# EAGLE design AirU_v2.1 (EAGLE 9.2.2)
COMPANY: ADAFRUIT INDUSTRIES; DRAWN: KTOWN; REV: B

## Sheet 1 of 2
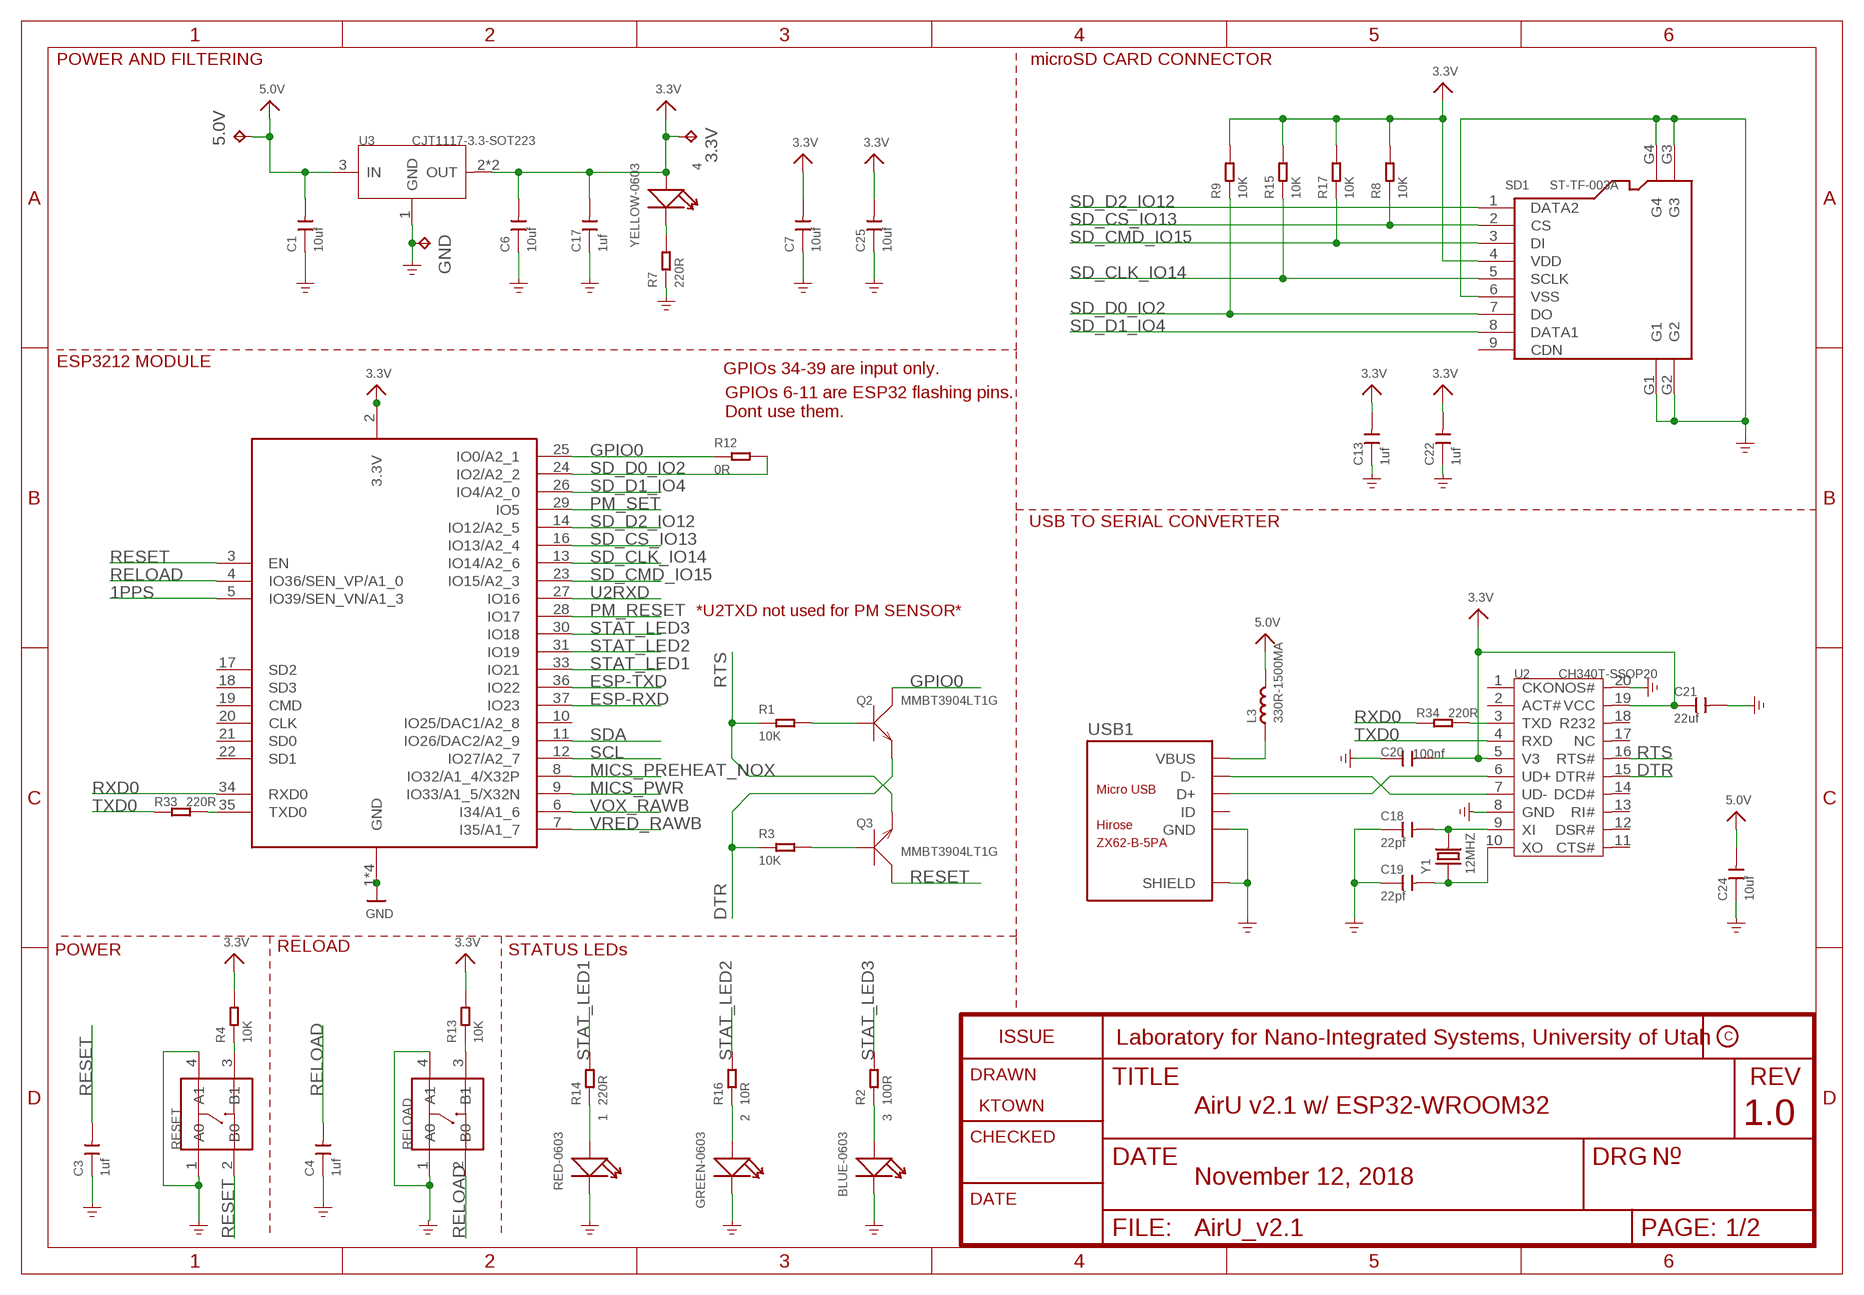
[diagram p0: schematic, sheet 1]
FRAME1 (FRAME_A4): COMPANY: TETRAD: SENSOR NETWORK SOLUTIONS, LLC; REV: 1.0

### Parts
1  RED-0603  LED-SMD-RED-DIFFUSED(0603)  [LED-0603]
2  GREEN-0603  SMD-LED-CLEAR-GREEN(0603)  [LED-0603]
3  BLUE-0603  SMD-LED-CLEAR-BLUE(0603)  [LED-0603]
3.3V  TPTP20SQ  [TP20SQ]
4  YELLOW-0603  SMD-LED-CLEAR-YELLOW(0603)  [LED-0603]
5.0V  TPTP20SQ  [TP20SQ]
C1  10uf  CERAMIC-10UF-10V-10%-X5R(0603)  [C0603]
C3  1uf  CERAMIC-1UF-25V-10%-X7R(0603)  [C0603]
C4  1uf  CERAMIC-1UF-25V-10%-X7R(0603)  [C0603]
C6  10uf  CERAMIC-10UF-10V-10%-X5R(0603)  [C0603]
C7  10uf  CERAMIC-10UF-10V-10%-X5R(0603)  [C0603]
C13  1uf  CERAMIC-1UF-25V-10%-X7R(0603)  [C0603]
C17  1uf  CERAMIC-1UF-25V-10%-X7R(0603)  [C0603]
C18  22pf  CERAMIC-22PF-50V-5%-NPO(0603)  [C0603]
C19  22pf  CERAMIC-22PF-50V-5%-NPO(0603)  [C0603]
C20  100nf  CERAMIC-100NF-50V-10%-X7R(0603)  [C0603]
C21  22uf  CERAMIC-22UF-6.3V-20%-X5R(0805)  [C0805]
C22  1uf  CERAMIC-1UF-25V-10%-X7R(0603)  [C0603]
C24  10uf  CERAMIC-10UF-10V-10%-X5R(0603)  [C0603]
C25  10uf  CERAMIC-10UF-10V-10%-X5R(0603)  [C0603]
GND  TPTP20SQ  [TP20SQ]
L3  330R-1500MA  SMD-FERRITE-BEAD-330R-1500MA(0805)'0805'  [L0805]
Q2  MMBT3904LT1G  SMD-TRANSISTORS-NPN-40V-200MA-MMBT3904LT1G(SOT-23)  [SOT-23]
Q3  MMBT3904LT1G  SMD-TRANSISTORS-NPN-40V-200MA-MMBT3904LT1G(SOT-23)  [SOT-23]
R1  10K  SMD-RES-10K-1%-1/10W(0603)  [R0603]
R2  100R  SMD-RES-100R-5%-1/10W(0603)  [R0603]
R3  10K  SMD-RES-10K-1%-1/10W(0603)  [R0603]
R4  10K  SMD-RES-10K-1%-1/10W(0603)  [R0603]
R7  220R  SMD-RES-220R-5%-1/10W(0603)  [R0603]
R8  10K  SMD-RES-10K-1%-1/10W(0603)  [R0603]
R9  10K  SMD-RES-10K-1%-1/10W(0603)  [R0603]
R12  0R  SMD-RES-0R-5%-1/10W(0603)  [R0603]
R13  10K  SMD-RES-10K-1%-1/10W(0603)  [R0603]
R14  220R  SMD-RES-220R-5%-1/10W(0603)  [R0603]
R15  10K  SMD-RES-10K-1%-1/10W(0603)  [R0603]
R16  10R  SMD-RES-10R-5%-1/10W(0603)  [R0603]
R17  10K  SMD-RES-10K-1%-1/10W(0603)  [R0603]
R33  220R  SMD-RES-220R-5%-1/10W(0603)  [R0603]
R34  220R  SMD-RES-220R-5%-1/10W(0603)  [R0603]
RELOAD  DIP-SWITCH-TACTILE-SPST-NO/TS-1109(4P-D6.0MM)'TS-1109'  [SW4-6.0X6.0X5.0MM]
RESET  DIP-SWITCH-TACTILE-SPST-NO/TS-1109(4P-D6.0MM)'TS-1109'  [SW4-6.0X6.0X5.0MM]
SD1  ST-TF-003A  MICRO-SD-CARD-SOCKET-9P(ST-TF-003A)  [MICRO-SD9+4P-SMD-16.1X14.5X1.85MM]
U2  CH340T-SSOP20  INTERFACE-CH340T(SSOP20)  [SSOP20-0.65-7.6X5.2MM]
U3  CJT1117-3.3-SOT223  PMIC-CJT1117-3.3(SOT223)  [SOT-223]
U7  ESP32_WROOM32_SKINNY  [WROOM32_SKINNY]
USB1  ZX62-B-5PA  MICRO-USB-SMD(ZX62-B-5PA)  [MICRO-USB5+6P-SMD-0.65-AB]
Y1  12MHZ  SMD-CRYSTAL-12MHZ-20PF-20PPM-40R(2P-5.0X3.2MM)  [X2-SMD-5.0X3.2X1.3MM]

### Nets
1PPS: U7.5(IO39/SEN_VN/A1_3) ; also sheet 2
3.3V: 3.3V.TP 4.+ C6.2 C7.2 C13.2 C17.2 C20.2 C21.1 C22.2 C25.2 R4.2 R8.2 R9.2 R13.2 R15.2 R17.2 SD1.4(VDD) U2.5(V3) U2.19(VCC) U3.2(OUT) U3.TER(OUT) U7.2(3.3V) ; also sheet 2
5.0V: 5.0V.TP C1.2 C24.2 L3.2 U3.3(IN) ; also sheet 2
DTR: Q2.2(E) R3.1 U2.15(DTR#)
ESP-RXD: U7.37(IO23) ; also sheet 2
ESP-TXD: U7.36(IO22) ; also sheet 2
GND: 1.- 2.- 3.- C1.1 C3.1 C4.1 C6.1 C7.1 C13.1 C17.1 C18.1 C19.1 C20.1 C21.2 C22.1 C24.1 C25.1 GND.TP R7.1 RELOAD.1(A0) RELOAD.4(A1) RESET.1(A0) RESET.4(A1) SD1.6(VSS) SD1.G1 SD1.G2 SD1.G3 SD1.G4 U2.8(GND) U2.20(NOS#) U3.1(GND) U7.1(GND) U7.15(GND) U7.38(GND) U7.P$1(GND) USB1.5(GND) USB1.P1(SHIELD) USB1.P2(SHIELD) USB1.P3_1(SHIELD) USB1.P3_2(SHIELD) USB1.P3_3(SHIELD) USB1.P4_1(SHIELD) USB1.P4_2(SHIELD) USB1.P4_3(SHIELD) USB1.P5(SHIELD) USB1.P6(SHIELD) ; supply symbol labelled GND_POWER ; also sheet 2
GPIO0: Q2.3(C) R12.1 U7.25(IO0/A2_1)
MICS_PREHEAT_NOX: U7.8(IO32/A1_4/X32P) ; also sheet 2
MICS_PWR: U7.9(IO33/A1_5/X32N) ; also sheet 2
N$1: 2.+ R16.1
N$7: 1.+ R14.1
N$12: Q3.1(B) R3.2
N$13: Q2.1(B) R1.2
N$22: 3.+ R2.1
N$25: 4.- R7.2
N$26: U2.7(UD-) USB1.2(D-)
N$27: U2.6(UD+) USB1.3(D+)
N$28: C18.2 U2.9(XI) Y1.2
N$29: C19.2 U2.10(XO) Y1.1
N$30: R34.2 U2.3(TXD)
N$33: R33.2 U7.35(TXD0)
N$37: R13.1 RELOAD.3(B1)
N$38: R4.1 RESET.3(B1)
PM_RESET: U7.28(IO17) ; also sheet 2
PM_SET: U7.29(IO5) ; also sheet 2
RELOAD: C4.2 RELOAD.2(B0) U7.4(IO36/SEN_VP/A1_0)
RESET: C3.2 Q3.3(C) RESET.2(B0) U7.3(EN)
RTS: Q3.2(E) R1.1 U2.16(RTS#)
RXD0: R34.1 U7.34(RXD0)
SCL: U7.12(IO27/A2_7) ; also sheet 2
SD_CLK_IO14: R15.1 SD1.5(SCLK) U7.13(IO14/A2_6)
SD_CMD_IO15: R17.1 SD1.3(DI) U7.23(IO15/A2_3)
SD_CS_IO13: R8.1 SD1.2(CS) U7.16(IO13/A2_4)
SD_D0_IO2: R9.1 R12.2 SD1.7(DO) U7.24(IO2/A2_2)
SD_D1_IO4: SD1.8(DATA1) U7.26(IO4/A2_0)
SD_D2_IO12: SD1.1(DATA2) U7.14(IO12/A2_5)
SDA: U7.11(IO26/DAC2/A2_9) ; also sheet 2
STAT_LED1: R14.2 U7.33(IO21)
STAT_LED2: R16.2 U7.31(IO19)
STAT_LED3: R2.2 U7.30(IO18)
TXD0: R33.1 U2.4(RXD)
U2RXD: U7.27(IO16) ; also sheet 2
VBUS: L3.1 USB1.1(VBUS)
VOX_RAWB: U7.6(I34/A1_6) ; also sheet 2
VRED_RAWB: U7.7(I35/A1_7) ; also sheet 2
Unconnected: SD1.9(CDN) U2.1(CKO) U2.2(ACT#) U2.11(CTS#) U2.12(DSR#) U2.13(RI#) U2.14(DCD#) U2.17(NC) U2.18(R232) U7.10(IO25/DAC1/A2_8) U7.17(SD2) U7.18(SD3) U7.19(CMD) U7.20(CLK) U7.21(SD0) U7.22(SD1) USB1.4(ID)

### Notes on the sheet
- POWER AND FILTERING | microSD CARD CONNECTOR
- ESP3212 MODULE
- GPIOs 34-39 are input only.
- GPIOs 6-11 are ESP32 flashing pins.
  Dont use them.
- USB TO SERIAL CONVERTER
- *U2TXD not used for PM SENSOR*
- POWER | RELOAD | STATUS LEDs
- Laboratory for Nano-Integrated Systems, University of Utah
- AirU v2.1 w/ ESP32-WROOM32
- November 12, 2018

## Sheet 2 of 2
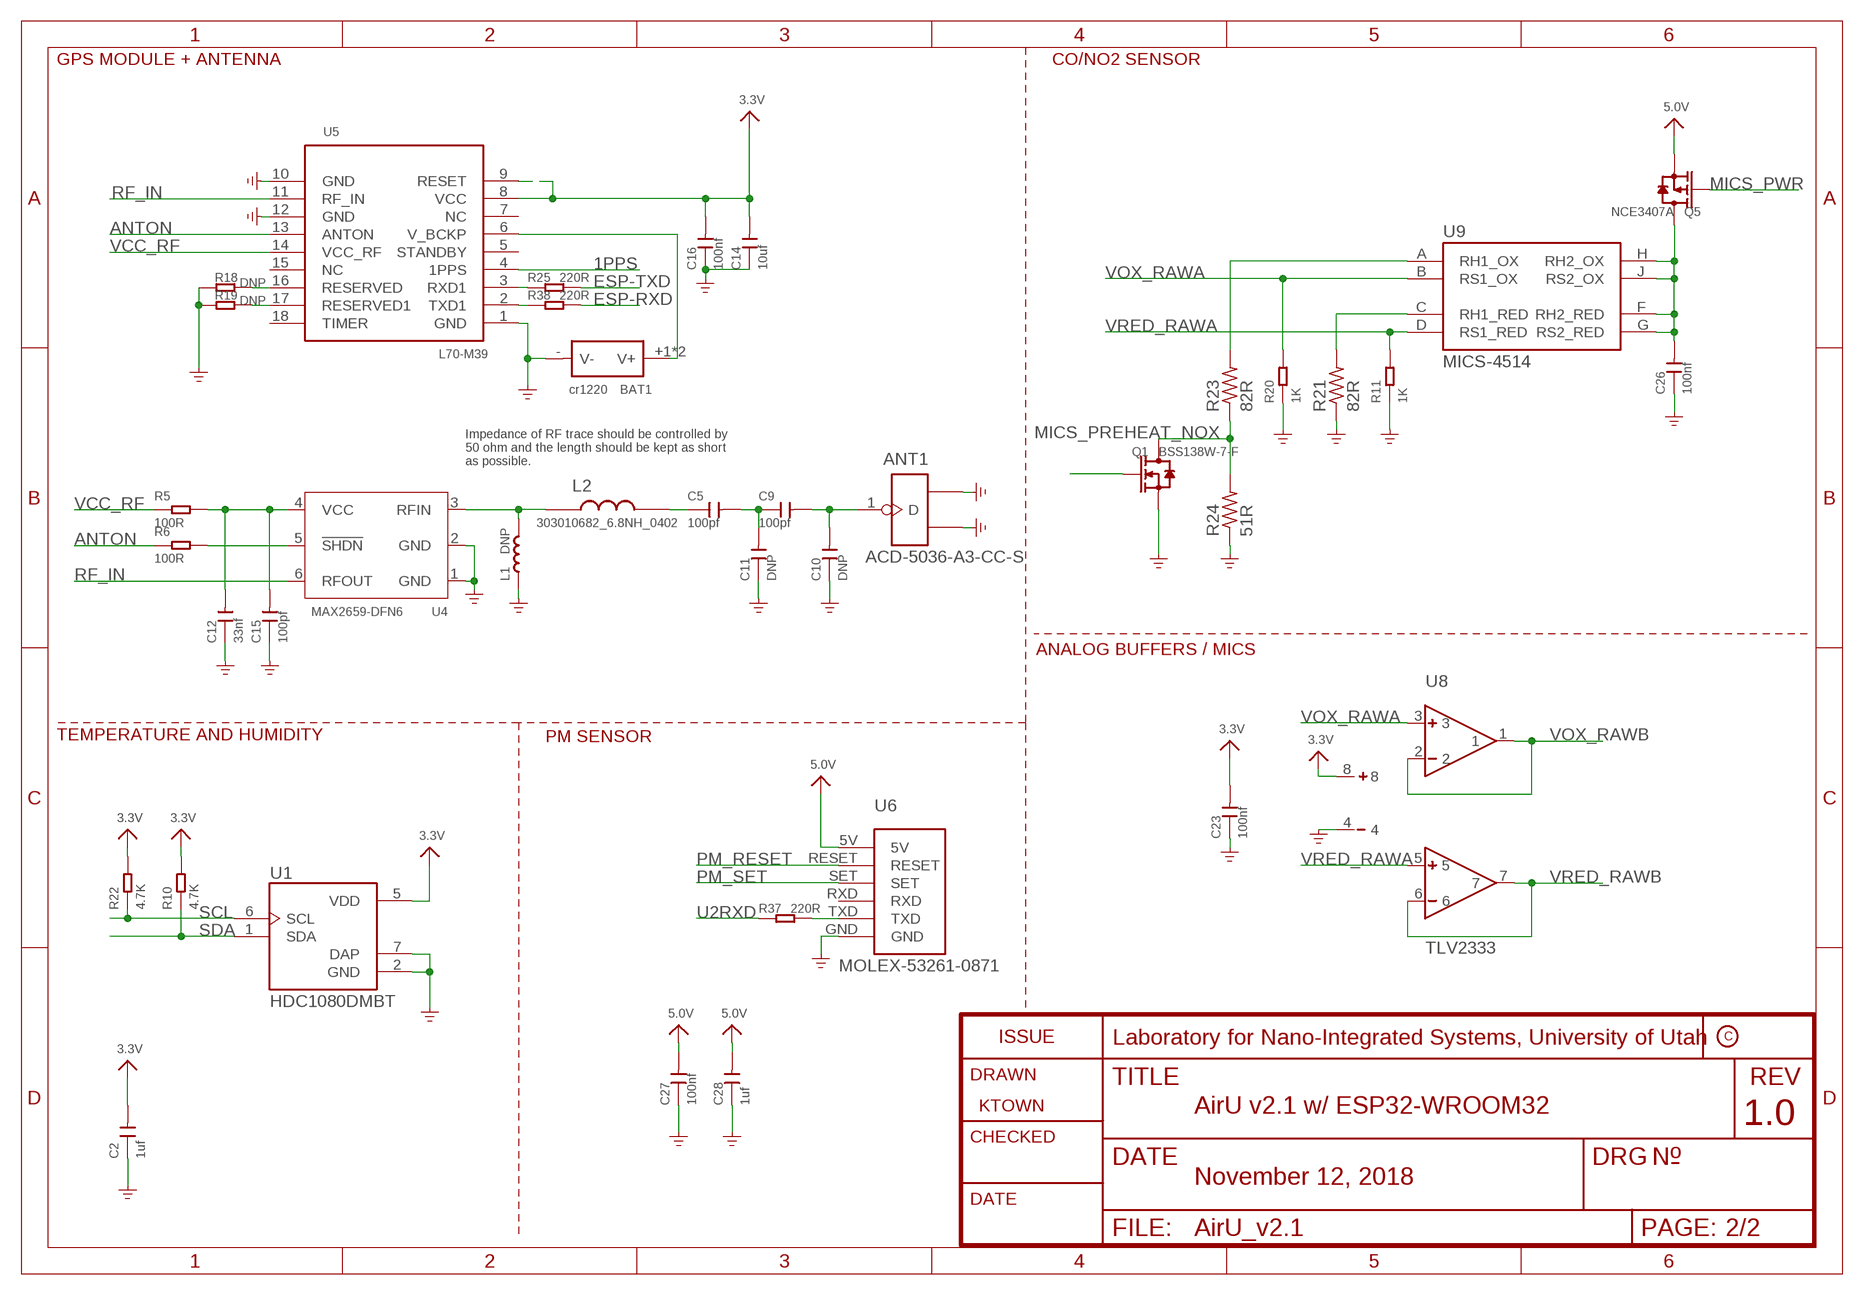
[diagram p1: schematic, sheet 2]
FRAME2 (FRAME_A4): COMPANY: TETRAD: SENSOR NETWORK SOLUTIONS, LLC; REV: 1.0
FRAME3 (FRAME_A4): COMPANY: TETRAD: SENSOR NETWORK SOLUTIONS, LLC; REV: 1.0

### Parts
ANT1  ACD-5036-A3-CC-S  ANTENNA-ACD5036  [ANT3-SMD-5.2X3.7X0.7MM]
BAT1  cr1220  DIP-BATTERY-CELL-HOLDER(1220)  [BAT2P-13.5-CR1220]
C2  1uf  CERAMIC-1UF-25V-10%-X7R(0603)  [C0603]
C5  100pf  CERAMIC-100PF-50V-5%-NPO(0603)  [C0603]
C9  100pf  CERAMIC-100PF-50V-5%-NPO(0603)  [C0603]
C10  DNP  CERAMIC-100PF-50V-5%-NPO(0603)  [C0603]
C11  DNP  CERAMIC-100PF-50V-5%-NPO(0603)  [C0603]
C12  33nf  CERAMIC-33NF-50V-10%-X7R(0603)  [C0603]
C14  10uf  CERAMIC-10UF-10V-10%-X5R(0603)  [C0603]
C15  100pf  CERAMIC-100PF-50V-5%-NPO(0603)  [C0603]
C16  100nf  CERAMIC-100NF-50V-10%-X7R(0603)  [C0603]
C23  100nf  CERAMIC-100NF-50V-10%-X7R(0603)  [C0603]
C26  100nf  CERAMIC-100NF-50V-10%-X7R(0603)  [C0603]
C27  100nf  CERAMIC-100NF-50V-10%-X7R(0603)  [C0603]
C28  1uf  CERAMIC-1UF-25V-10%-X7R(0603)  [C0603]
L1  DNP  INDUCTOR/FERRITE-BEAD-0201  [L0201]
L2  303010682_6.8NH_0402  [L0402]
Q1  BSS138W-7-F  SMD-MOSFET-N-CH-50V-200MA-BSS138W-7-F(SOT-23)  [SOT-23]
Q5  NCE3407A  SMD-MOSFET-P-CH-VDC=30V-ID=4.3A-NCE3407A(SOT-23)  [SOT-23]
R5  100R  SMD-RES-100R-5%-1/10W(0603)  [R0603]
R6  100R  SMD-RES-100R-5%-1/10W(0603)  [R0603]
R10  4.7K  SMD-RES-4.7K-5%-1/10W(0603)  [R0603]
R11  1K  SMD-RES-1K-1%-1/10W(0603)  [R0603]
R18  DNP  SMD-RES-10K-1%-1/10W(0603)  [R0603]
R19  DNP  SMD-RES-10K-1%-1/10W(0603)  [R0603]
R20  1K  SMD-RES-1K-1%-1/10W(0603)  [R0603]
R21  82R  R-US_R0603  [R0603]
R22  4.7K  SMD-RES-4.7K-5%-1/10W(0603)  [R0603]
R23  82R  R-US_R0603  [R0603]
R24  51R  R-US_R0603  [R0603]
R25  220R  SMD-RES-220R-5%-1/10W(0603)  [R0603]
R37  220R  SMD-RES-220R-5%-1/10W(0603)  [R0603]
R38  220R  SMD-RES-220R-5%-1/10W(0603)  [R0603]
U1  HDC1080DMBT  [SON100P300X300X80-7N]
U4  MAX2659-DFN6  AMPLIFIER-MAX2659  [DFN6-0.5-1.5X1.2X0.72MM]
U5  L70-M39  MOUDLE-GPS-L70-HARDWARE  [LGA18-1.1-9.7X10.1X2.5MM]
U6  MOLEX-53261-0871  [MOLEX-53261-0871]
U8  TLV2333  [TLV2333]
U9  MICS-4514  [MICS_10-SMD]

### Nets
1PPS: U5.4(1PPS) ; also sheet 1
3.3V: C2.2 C14.2 C16.2 C23.2 R10.2 R22.2 U1.5(VDD) U5.8(VCC) U5.9(RESET) U8.8 ; also sheet 1
5.0V: C27.2 C28.2 Q5.2(S) U6.5V ; also sheet 1
ANTON: R6.1 U5.13(ANTON)
ESP-RXD: R38.2 ; also sheet 1
ESP-TXD: R25.2 ; also sheet 1
GND: ANT1.2(GND1) ANT1.3(GND2) BAT1.-(V-) C2.1 C10.1 C11.1 C12.1 C14.1 C15.1 C16.1 C23.1 C26.1 C27.1 C28.1 L1.1 Q1.2(S) R11.1 R18.1 R19.1 R20.1 R21.1 R24.1 U1.2(GND) U1.7(DAP) U4.1(GND) U4.2(GND) U5.1(GND) U5.10(GND) U5.12(GND) U6.GND U8.4 ; supply symbol labelled GND_POWER ; also sheet 1
MICS_PREHEAT_NOX: Q1.1(G) ; also sheet 1
MICS_PWR: Q5.1(G) ; also sheet 1
N$2: R21.2 U9.C(RH1_RED)
N$3: C5.2 C9.1 C11.2
N$4: ANT1.1(D) C9.2 C10.2
N$5: L1.2 L2.P$1 U4.3(RFIN)
N$6: R23.2 U9.A(RH1_OX)
N$8: C5.1 L2.P$2
N$9: R6.2 U4.5(!SHDN)
N$10: C12.2 C15.2 R5.2 U4.4(VCC)
N$11: R18.2 U5.16(RESERVED)
N$14: R19.2 U5.17(RESERVED1)
N$23: Q1.3(D) R23.1 R24.2
N$24: C26.2 Q5.3(D) U9.F(RH2_RED) U9.G(RS2_RED) U9.H(RH2_OX) U9.J(RS2_OX)
N$36: R37.2 U6.TXD
PM_RESET: U6.RESET ; also sheet 1
PM_SET: U6.SET ; also sheet 1
RF_IN: U4.6(RFOUT) U5.11(RF_IN)
SCL: R22.1 U1.6(SCL) ; also sheet 1
SDA: R10.1 U1.1(SDA) ; also sheet 1
U1RXD: R25.1 U5.3(RXD1)
U1TXD: R38.1 U5.2(TXD1)
U2RXD: R37.1 ; also sheet 1
V_BCKP: BAT1.+1(V+) BAT1.+2(V+) U5.6(V_BCKP)
VCC_RF: R5.1 U5.14(VCC_RF)
VOX_RAWA: R20.2 U8.3 U9.B(RS1_OX)
VOX_RAWB: U8.1 U8.2 ; also sheet 1
VRED_RAWA: R11.2 U8.5 U9.D(RS1_RED)
VRED_RAWB: U8.6 U8.7 ; also sheet 1
Unconnected: U5.5(STANDBY) U5.7(NC) U5.15(NC) U5.18(TIMER) U6.RXD

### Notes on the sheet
- GPS MODULE + ANTENNA | CO/NO2 SENSOR
- Impedance of RF trace should be controlled by 
  50 ohm and the length should be kept as short 
  as possible.
- ANALOG BUFFERS / MICS
- TEMPERATURE AND HUMIDITY | PM SENSOR
- Laboratory for Nano-Integrated Systems, University of Utah
- AirU v2.1 w/ ESP32-WROOM32
- November 12, 2018

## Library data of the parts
1 = Seeed-LED:LED-SMD-RED-DIFFUSED(0603): 304090042; MPN: 19-217-R6C-AL1M2VY-3T
2 = Seeed-LED:SMD-LED-CLEAR-GREEN(0603): 304090043; MPN: 19-217-G7C-AN1P2-3T
3 = Seeed-LED:SMD-LED-CLEAR-BLUE(0603): 304090045; MPN: 19-217-BHC-ZL1M2RY-3T
3.3V 5.0V GND = testpad:TP: Test pad
4 = Seeed-LED:SMD-LED-CLEAR-YELLOW(0603): 304090044; MPN: 19-217-Y5C-AM1N1VY-3T
ANT1 = Connector-new:ANTENNA-ACD5036; MPN: ACD-5036-A3-CC-S
BAT1 = Seeed-Connector:DIP-BATTERY-CELL-HOLDER(1220): 320170002
C1 C6 C7 C14 C24 C25 = Seeed-Capacitor:CERAMIC-10UF-10V-10%-X5R(0603): 302010103; MPN: CC0603KRX5R6BB106
C2-C4 C13 C17 C22 C28 = Seeed-Capacitor:CERAMIC-1UF-25V-10%-X7R(0603): 302010139; MPN: CC0603KRX7R8BB105
C5 C9 C15 = Seeed-Capacitor:CERAMIC-100PF-50V-5%-NPO(0603): 302010076; MPN: CC0603JRNPO9BN101
C10 C11 = Seeed-Capacitor:CERAMIC-100PF-50V-5%-NPO(0603): 302010076; MPN: CC0603JRNPO9BN101; VALUE: 100pf
C12 = Seeed-Capacitor:CERAMIC-33NF-50V-10%-X7R(0603): 302010088; MPN: CC0603KRX7R9BB333
C16 C20 C23 C26 C27 = Seeed-Capacitor:CERAMIC-100NF-50V-10%-X7R(0603): 302010138; MPN: CC0603KRX7R9BB104
C18 C19 = Seeed-Capacitor:CERAMIC-22PF-50V-5%-NPO(0603): 302010143; MPN: CC0603JRNPO9BN220
C21 = Seeed-Capacitor:CERAMIC-22UF-6.3V-20%-X5R(0805): 302010171; MPN: CC0805MKX5R5BB226
L1 = Discrete-new:INDUCTOR/FERRITE-BEAD
L2 = Seeed-OPL-2017-01-Inductor-Akita:303010682_6.8NH_0402: Murata;LQW15AN6N8G00D, SMD Inductor 6.8nH-2%-700mA;0402, SKU: 303010682
L3 = Seeed-Inductor:SMD-FERRITE-BEAD-330R-1500MA(0805): 303030006; MPN: BLM21PG331SN1D
Q1 = Seeed-Transistor:SMD-MOSFET-N-CH-50V-200MA-BSS138W-7-F(SOT-23): 305030000; MPN: BSS138W-7-F
Q2 Q3 = Seeed-Transistor:SMD-TRANSISTORS-NPN-40V-200MA-MMBT3904LT1G(SOT-23): 305010013; MPN: MMBT3904LT1G
Q5 = Seeed-Transistor:SMD-MOSFET-P-CH-VDC=30V-ID=4.3A-NCE3407A(SOT-23): 305030010; MPN: NCE3407A
R1 R3 R4 R8 R9 R13 R15 R17 = Seeed-Resistor:SMD-RES-10K-1%-1/10W(0603): 301010299; MPN: RC0603FR-0710KL
R2 R5 R6 = Seeed-Resistor:SMD-RES-100R-5%-1/10W(0603): 301010090; MPN: RC0603JR-07100RL
R7 R14 R25 R33 R34 R37 R38 = Seeed-Resistor:SMD-RES-220R-5%-1/10W(0603): 301010163; MPN: RC0603JR-07220RL
R10 R22 = Seeed-Resistor:SMD-RES-4.7K-5%-1/10W(0603): 301010290; MPN: RC0603JR-074K7L
R11 R20 = Seeed-Resistor:SMD-RES-1K-1%-1/10W(0603): 301010298; MPN: RC0603FR-071KL
R12 = Seeed-Resistor:SMD-RES-0R-5%-1/10W(0603): 301010292; MPN: RC0603JR-070RL
R16 = Seeed-Resistor:SMD-RES-10R-5%-1/10W(0603): 301010096; MPN: RC0603JR-0710RL
R18 R19 = Seeed-Resistor:SMD-RES-10K-1%-1/10W(0603): 301010299; MPN: RC0603FR-0710KL; VALUE: 10K
R21 R23 R24 = rcl:R-US_: RESISTOR, American symbol; SPICEPREFIX: R
RELOAD RESET = Seeed-Switch:DIP-SWITCH-TACTILE-SPST-NO/TS-1109(4P-D6.0MM): 311020024
SD1 = Seeed-Connector:MICRO-SD-CARD-SOCKET-9P(ST-TF-003A): 320090000; MPN: ST-TF-003A
U1 = HDC1080DMBT_TITempHum:HDC1080DMBT: HDC1080 Low Power, High Accuracy Digital Humidity Sensor with Temperature Sensor 6-WSON -40 to 125; DESCRIPTION: HDC1080 Low Power, High Accuracy Digital Humidity Sensor with Temperature Sensor 6-WSON -40 to 125; DIGI-KEY_PART_NUMBER: 296-43864-1-ND; DIGI-KEY_PURCHASE_URL: https://www.digikey.com/product-detail/en/texas-instruments/HDC1080DMBT/296-43864-1-ND/5878615?utm_source=snapeda&utm_medium=aggregator&utm_campaign=symbol; MF: Texas Instruments; MP: HDC1080DMBT; PACKAGE: WDFN-6 Texas Instruments
U2 = Seeed-IC:INTERFACE-CH340T(SSOP20): 310070026; MPN: CH340T
U3 = Seeed-IC:PMIC-CJT1117-3.3(SOT223): 310030097; MPN: CJT1117-3.3
U4 = IC-new:AMPLIFIER-MAX2659: GPS/GNSS Low-Noise Amplifier; MPN: MAX2659
U5 = moudle-new:MOUDLE-GPS-L70-HARDWARE: L70 GPS module; MPN: L70; VALUE: L70
U6 = Molex_53261_0871_Connector:MOLEX-53261-0871
U7 = microbuilder:ESP32_WROOM32
U8 = tlv2333:TLV2333
U9 = MICS-4514:MICS-4514: Metal oxide MEMS carbon monoxide (CO) and NOx sensor in an SMD package.; AVAILABILITY: Unavailable; MF: Amphenol; MP: MICS-4514; PACKAGE: None; PRICE: 11.82 USD
USB1 = Seeed-Connector:MICRO-USB-SMD(ZX62-B-5PA): 320010005; MPN: ZX62-B-5PA
Y1 = Seeed-Crystal Oscillator:SMD-CRYSTAL-12MHZ-20PF-20PPM-40R(2P-5.0X3.2MM): 306010047; MPN: 5032/2P

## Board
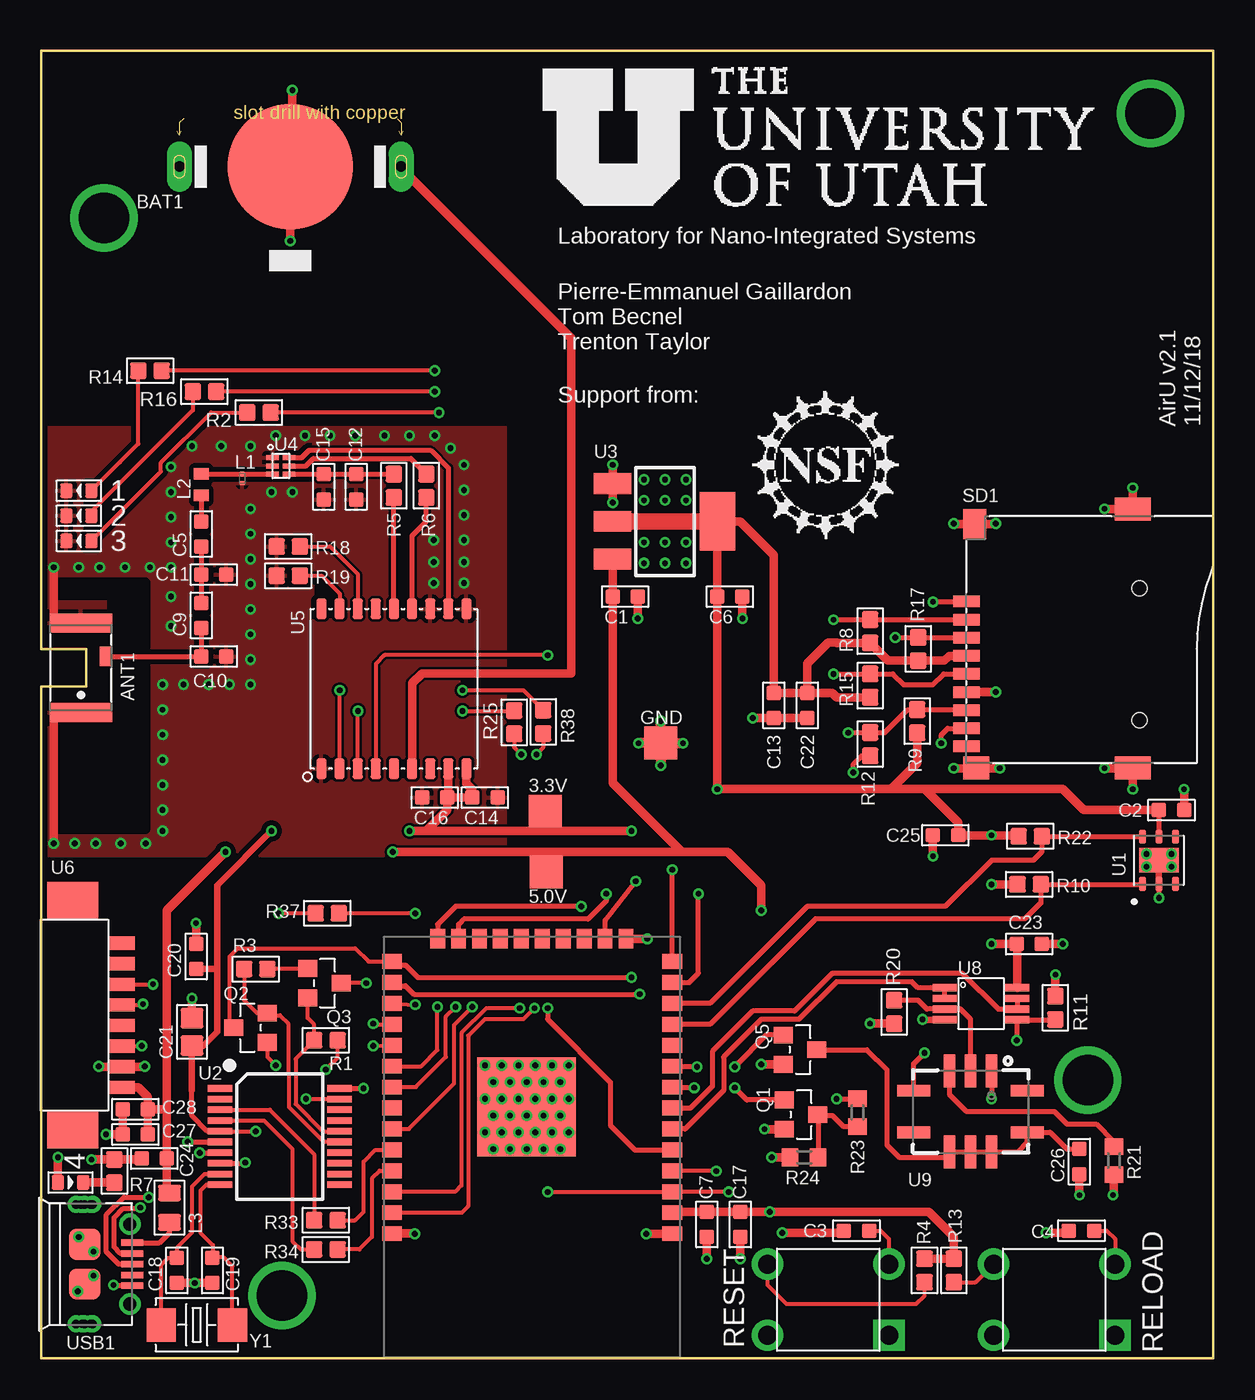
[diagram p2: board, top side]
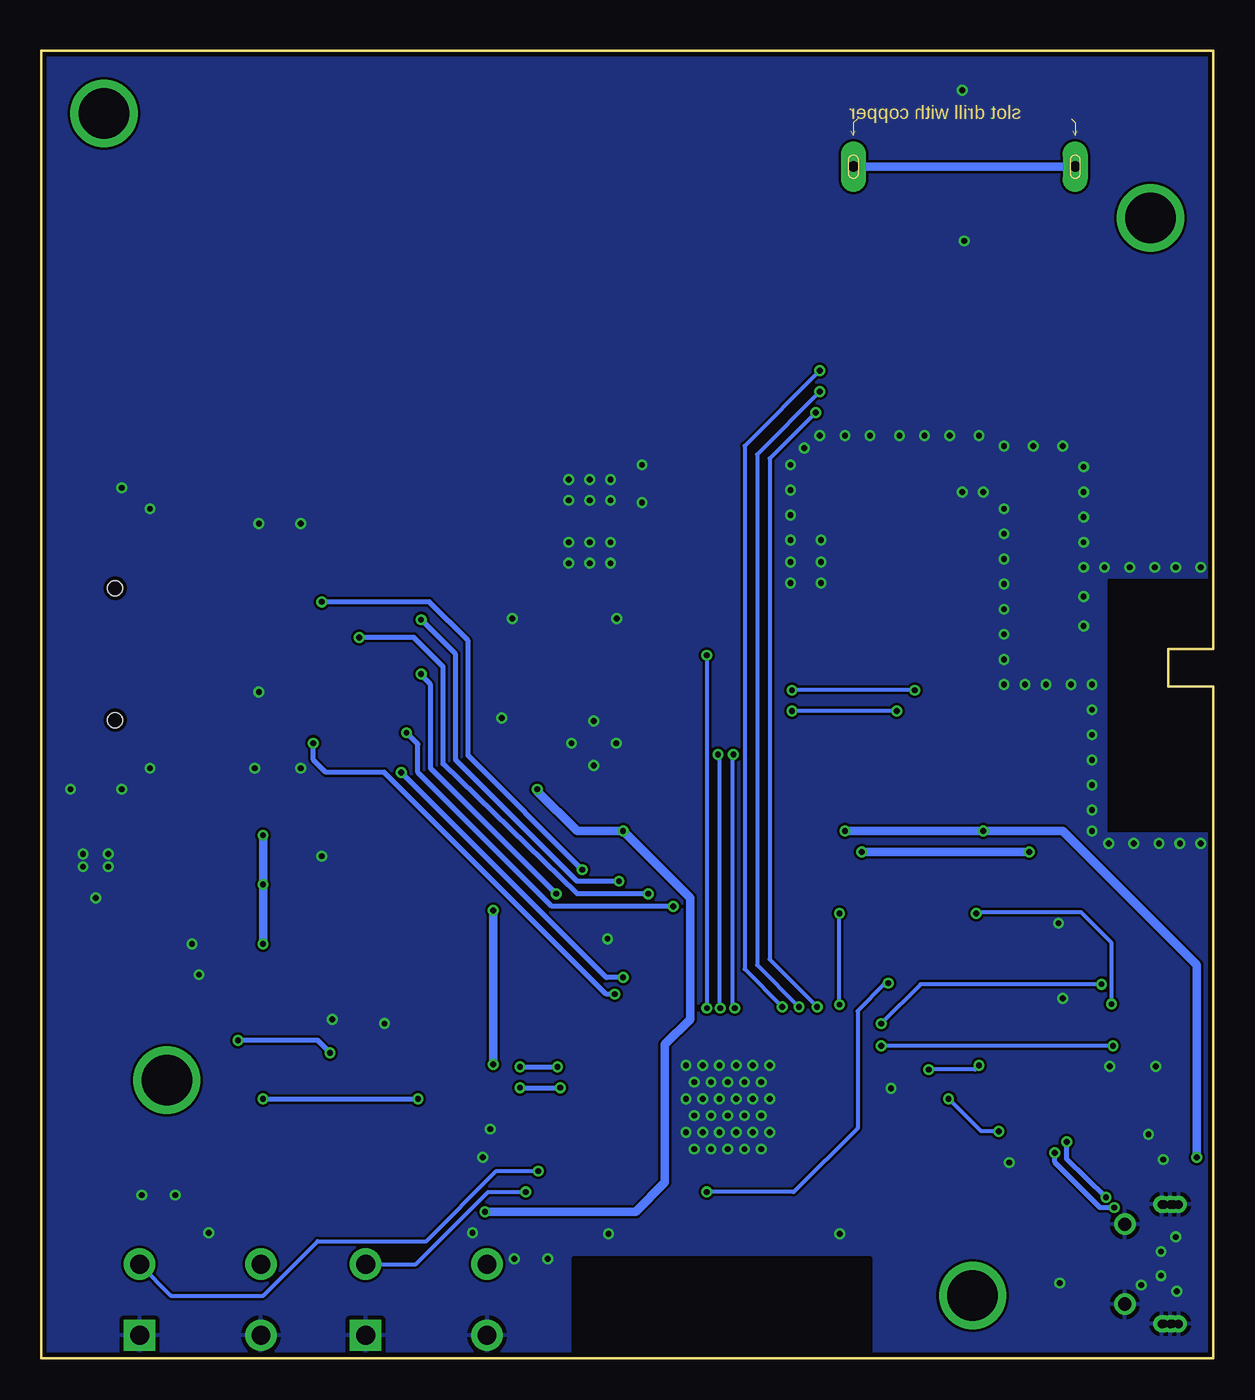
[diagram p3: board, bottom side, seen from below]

Size 71.12 x 79.38 mm. Coordinates in mm from the lower left corner, seen from the top.
Outline: 0,0 71.12,0 71.12,79.38 0,79.38 0,43.05 2.73,43.05 2.73,40.77 0,40.77 0,0
Copper layers (1*16): Top 0.035mm / dielectric 1.5mm / Bottom 0.035mm
Design rules "SeeedStudio_2layer_DRU_no_angle_20140221": minimum track width 6mil, minimum drill 12mil, track to track 6mil, track to pad 6mil, pad to pad 6mil, via to via 6mil, smd to smd 0mil, copper to edge 10mil, drill to drill 10mil, minimum pad ring 10mil, minimum via ring 6mil, stop-mask expansion 2mil, vias tented up to drill 100mil, thermal gap 10mil
tRestrict: area 20.8,0.1 to 38.8,6.1
bRestrict: area 20.8,0.1 to 38.8,6.1; area 0,32.1 to 6.3,47.1; area 0,32 to 6.3,47.2

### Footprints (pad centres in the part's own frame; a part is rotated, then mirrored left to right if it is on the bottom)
LED-0603 = smd 0.762 x 0.889: + -0.762,0; - 0.762,0
TP20SQ = smd 2 x 2: TP 0,0
ANT3-SMD-5.2X3.7X0.7MM = smd 0.75 x 1.2: 1 1.525,0.7 | smd 3.8 x 1.15: 2 0,2.725; 3 0,-2.725
BAT2P-13.5-CR1220 = drill 0.635 pad 1.524 long: +1 6.731,0; +2 -6.731,0 | smd 7.62 x 7.62: - 0,0
C0603 = smd 0.889 x 0.889: 1 0,0.762; 2 0,-0.762
C0805 = smd 1.397 x 1.27: 1 0,0.835; 2 0,-0.835
L0201 = smd 0.279 x 0.318: 1 -0.279,0; 2 0.279,0
L0402 = smd 0.7 x 0.9: P$1 -0.65,0; P$2 0.65,0
L0805 = smd 1.016 x 1.397: 1 -0.889,0; 2 0.889,0
SOT-23 = smd 1.016 x 1.143: 1 -0.889,-1.016; 2 0.889,-1.016; 3 0,1.016
R0603 = smd 1.016 x 1.016: 1 0,0.708; 2 0,-0.708
R0603' = smd 1 x 1.1: 1 -0.85,0; 2 0.85,0
SW4-6.0X6.0X5.0MM = drill 1.143 pad 1.905 square: 1 -3.683,2.159 | drill 1.143 pad 1.905: 2 -3.683,-2.159; 3 3.683,-2.159; 4 3.683,2.159
MICRO-SD9+4P-SMD-16.1X14.5X1.85MM = smd 1.6 x 0.7: 1 0,2.25; 2 0,1.15; 3 0,0.05; 4 0,-1.05; 5 0,-2.15; 6 0,-3.25; 7 0,-4.35; 8 0,-5.45; 9 0,-6.55 | smd 1.6 x 1.4: G1 0.6,-7.85 | smd 2.2 x 1.4: G2 10.1,-7.85; G3 10.1,7.85 | smd 1.4 x 1.8: G4 0.5,6.95 | hole 0.9: 10.5,-4.95; 10.5,3.05
SON100P300X300X80-7N = smd 0.86 x 0.42: 1 -1.435,1; 2 -1.435,0; 3 -1.435,-1; 4 1.435,-1; 5 1.435,0; 6 1.435,1 | smd 1.5 x 2.4: 7 0,0
SSOP20-0.65-7.6X5.2MM = smd 0.4 x 1.5: 1 -2.925,-3.625; 2 -2.275,-3.625; 3 -1.625,-3.625; 4 -0.975,-3.625; 5 -0.325,-3.625; 6 0.325,-3.625; 7 0.975,-3.625; 8 1.625,-3.625; 9 2.275,-3.625; 10 2.925,-3.625; 11 2.925,3.625; 12 2.275,3.625; 13 1.625,3.625; 14 0.975,3.625; 15 0.325,3.625; 16 -0.325,3.625; 17 -0.975,3.625; 18 -1.625,3.625; 19 -2.275,3.625; 20 -2.925,3.625
SOT-223 = smd 1.27 x 2.286: 1 -2.286,-3.175; 2 0,-3.175; 3 2.286,-3.175 | smd 3.556 x 2.159: TER 0,3.175
DFN6-0.5-1.5X1.2X0.72MM = smd 0.3 x 0.75: 1 -0.5,-0.5; 2 0,-0.5; 3 0.5,-0.5; 4 0.5,0.5; 5 0,0.5; 6 -0.5,0.5
LGA18-1.1-9.7X10.1X2.5MM = smd 1.27 x 0.635: 1 4.85,-4.4; 2 4.85,-3.3; 3 4.85,-2.2; 4 4.85,-1.1; 5 4.85,0; 6 4.85,1.1; 7 4.85,2.2; 8 4.85,3.3; 9 4.85,4.4; 10 -4.85,4.4; 11 -4.85,3.3; 12 -4.85,2.2; 13 -4.85,1.1; 14 -4.85,0; 15 -4.85,-1.1; 16 -4.85,-2.2; 17 -4.85,-3.3; 18 -4.85,-4.4
MOLEX-53261-0871 = smd 0.8 x 1.6: 5V 4.375,0.8; GND 3.125,0.8; NC@1 -4.375,0.8; NC@2 -3.125,0.8; RESET -1.875,0.8; RXD 0.625,0.8; SET 1.875,0.8; TXD -0.625,0.8 | smd 2.2 x 3.1: NC@3 -6.975,-2.16; NC@4 6.975,-2.16
WROOM32_SKINNY = smd 1.2 x 0.9: 1 -8.5,5; 2 -8.5,3.73; 3 -8.5,2.46; 4 -8.5,1.19; 5 -8.5,-0.08; 6 -8.5,-1.35; 7 -8.5,-2.62; 8 -8.5,-3.89; 9 -8.5,-5.16; 10 -8.5,-6.43; 11 -8.5,-7.7; 12 -8.5,-8.97; 13 -8.5,-10.24; 14 -8.5,-11.51; 25 8.5,-11.51; 26 8.5,-10.24; 27 8.5,-8.97; 28 8.5,-7.7; 29 8.5,-6.43; 30 8.5,-5.16; 31 8.5,-3.89; 32 8.5,-2.62; 33 8.5,-1.35; 34 8.5,-0.08; 35 8.5,1.19; 36 8.5,2.46; 37 8.5,3.73; 38 8.5,5 | smd 0.9 x 1.2: 15 -5.7,-12.9; 16 -4.43,-12.9; 17 -3.16,-12.9; 18 -1.89,-12.9; 19 -0.62,-12.9; 20 0.65,-12.9; 21 1.92,-12.9; 22 3.19,-12.9; 23 4.46,-12.9; 24 5.73,-12.9 | smd 6 x 6: P$1 0.34,-2.7
TLV2333 = smd 1.45 x 0.45: 1 0.725,2.175; 2 0.725,1.525; 3 0.725,0.875; 4 0.725,0.225; 5 5.125,0.225; 6 5.125,0.875; 7 5.125,1.525; 8 5.125,2.175
MICS_10-SMD = smd 0.7 x 2: A 1.27,2.45; B 0,2.45; C -1.27,2.45; F -1.27,-2.45; G 0,-2.45; H 1.27,-2.45 | smd 2 x 0.7: D -3.45,1.27; E -3.45,-1.27; J 3.45,-1.27; K 3.45,1.27
MICRO-USB5+6P-SMD-0.65-AB = smd 0.4 x 1.35: 1 -1.3,2.875; 2 -0.65,2.875; 3 0,2.875; 4 0.65,2.875; 5 1.3,2.875 | smd 1.9 x 1.9: P1 -1.2,0; P2 1.2,0 | drill 0.508 pad 1.016: P3_1 -3.625,-0.533; P3_2 -3.625,-0.025; P3_3 -3.625,0.483; P4_1 3.625,-0.533; P4_2 3.625,-0.025; P4_3 3.625,0.483 | drill 0.8: P5 -2.425,2.73; P6 2.425,2.73
X2-SMD-5.0X3.2X1.3MM = smd 1.778 x 2.032: 1 -2.159,0; 2 2.159,0

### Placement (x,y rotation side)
1  2.29,52.66 180 top
2  2.29,51.14 180 top
3  2.29,49.61 180 top
3.3V  30.58,33.21 0 top
4  1.78,10.67 0 top
5.0V  30.65,29.52 0 top
ANT1  2.41,41.91 0 top
BAT1  15.11,72.33 180 top
C1  35.43,46.23 270 top
C2  68.58,33.27 270 top
C3  49.47,7.75 90 top
C4  63.12,7.75 90 top
C5  9.72,50.04 0 top
C6  41.78,46.23 270 top
C7  40.39,8.13 180 top
C9  9.72,45.09 0 top
C10  10.48,42.61 270 top
C11  10.48,47.56 270 top
C12  19.11,52.9 180 top
C13  44.45,39.62 180 top
C14  26.92,34.04 270 top
C15  17.14,52.9 180 top
C16  23.88,34.04 90 top
C17  42.42,8.13 180 top
C18  8.23,5.33 180 top
C19  10.39,5.33 180 top
C20  9.4,24.38 0 top
C21  9.14,19.81 180 top
C22  46.48,39.62 180 top
C23  59.94,25.15 270 top
C24  6.86,12.13 90 top
C25  54.86,31.75 90 top
C26  62.99,11.94 180 top
C27  5.71,13.59 90 top
C28  5.71,15.11 90 top
GND  37.59,37.33 0 top
L1  12.19,53.4 90 top
L2  9.72,53.02 270 top
L3  7.79,9.14 90 top
Q1  46.1,14.8 270 top
Q2  12.7,20.07 90 top
Q3  17.18,22.77 270 top
Q5  46.04,18.73 270 top
R1  17.27,19.3 90 top
R2  13.21,57.4 90 top
R3  13.02,23.62 90 top
R4  53.59,5.33 180 top
R5  21.4,52.96 180 top
R6  23.37,52.96 180 top
R7  4.45,11.37 0 top
R8  50.29,44.13 0 top
R9  53.15,38.67 0 top
R10  59.94,28.77 270 top
R11  61.53,21.27 0 top
R12  50.29,37.27 180 top
R13  55.37,5.33 180 top
R14  6.6,59.94 90 top
R15  50.29,40.83 0 top
R16  9.91,58.67 90 top
R17  53.21,43.05 0 top
R18  14.99,49.28 90 top
R19  14.99,47.5 90 top
R20  51.75,21.02 180 top
R21  82R  [R0603']  65.09,12 90 top
R22  60.01,31.69 270 top
R23  82R  [R0603']  49.53,14.92 90 top
R24  51R  [R0603']  46.29,12.19 0 top
R25  28.7,38.6 0 top
R33  17.27,6.6 90 top
R34  17.27,8.38 270 top
R37  17.36,27.01 270 top
R38  30.46,38.63 0 top
RELOAD  61.47,3.56 180 top
RESET  47.75,3.56 180 top
SD1  56.13,43.69 0 top
U1  67.82,30.23 90 top
U2  14.48,13.46 270 top
U3  37.85,50.8 270 top
U4  14.54,54.17 270 top
U5  21.4,40.64 270 top
U6  4.06,20.83 270 top
U7  29.78,12.57 180 top
U8  54.1,20.32 0 top
U9  56.39,14.99 0 top
USB1  2.65,5.71 270 top
Y1  9.44,2.03 180 top

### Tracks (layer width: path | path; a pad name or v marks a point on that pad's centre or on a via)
1PPS  (via drill 0.35)
  Top 0.254: v30.73,42.67 | v30.73,42.67 20.83,42.67 20.3,42.14 U5.4
  Top 0.305: v30.73,21.25 30.73,20.57 34.54,16.76 34.54,14.14 36.02,12.65 U7.5
  Bottom 0.254: v30.73,42.67 v30.73,21.25
3.3V  (via drill 0.35)
  Top 0.254: U2.5 v13.01,13.79 v13.02,13.78 | v16.07,15.75 U2.19
  Top 0.305: C2.2 U1.5 | U2.5 10.09,13.79 9.14,14.73 9.14,16.26
  Top 0.406: 9.14,16.26 C21.1 9.83,18.98 10.67,19.81 10.67,23.62 | v13.97,32 10.67,28.7 10.67,23.62 | 10.67,23.62 C20.2
  Top 0.508: 23.37,32 v22.35,32 | U5.8 24.7,34.1 C16.2 | SD1.4 55.08,42.64 54.79,42.34 R17.2 51.37,42.34 R8.2 48.27,43.42 48.26,43.43 47.75,43.43 46.48,42.16 C22.2 | C16.2 24.64,33.27 23.37,32 | 51.56,34.54 53.59,34.54 | 53.59,34.54 61.98,34.54 63.25,33.27 C2.2 | 51.56,34.54 53.15,36.13 R9.2 | R4.2 R13.2 55.37,7.37 53.85,8.89 v44.2,8.89 C17.2 C7.2 38.33,8.89 U7.2 | C22.2 C13.2 44.45,48.77 42.42,50.8 U3.TER C6.2 v41.02,34.54 51.56,34.54 | C22.2 48.01,40.39 48.27,40.12 R15.2 | 23.37,32 30.22,32 | 30.22,32 30.58,32 | 30.58,32 31.15,32 | 31.15,32 v35.81,32 | 53.59,34.54 55.63,32.51 C25.2 v57.66,31.75 59.24,31.75 R22.2 | v57.66,28.77 R10.2 | v57.66,25.15 C23.2 59.23,25.1 U8.8 | v1.02,12.19 4.+ | C16.2 C14.2 26.16,34.54 25.8,34.9 U5.9 | 30.58,32 3.3V.TP | 3.3V.TP 30.58,33.12 30.22,32.76 30.22,32 | 3.3V.TP 30.6,33.19 31.15,33.19 31.15,32
  Top 1.016: U3.2 U3.TER
  Bottom 0.152: v1.02,12.19
  Bottom 0.254: v13.02,13.78 14.1,13.78 v16.07,15.75
  Bottom 0.508: v22.35,32 v13.97,32 9.14,32 1.02,23.88 v1.02,12.19 | v44.2,8.89 35.05,8.89 33.27,10.67 33.27,19.05 31.75,20.57 31.75,27.94 v35.81,32 38.61,32 41.02,34.42 v41.02,34.54 | v57.66,31.75 v57.66,28.77 v57.66,25.15 | v1.02,12.19
5.0V  (via drill 0.35)
  Top 0.508: v21.34,30.73 29.97,30.73 | 31.24,30.73 31.75,30.73 38.86,30.73 | 38.86,30.73 41.66,30.73 43.69,28.7 v43.69,27.18 | v11.18,30.73 7.62,27.18 7.62,15.11 | 38.86,30.73 34.67,34.92 C1.2 U3.3 | C28.2 6.48,15.88 5.9,16.45 U6.5V | C28.2 C27.2 | C28.2 7.62,15.11 | 7.62,15.11 C24.2 7.62,10.2 L3.2 | v43.69,17.84 Q5.2 | 29.97,30.73 30.65,30.06 5.0V.TP 30.65,30.14 31.24,30.73 | 29.97,30.73 31.24,30.73
  Bottom 0.508: v11.18,30.73 v21.34,30.73 | v43.69,27.18 v43.69,17.84
ANTON
  Top 0.305: U5.13 22.5,49.93 23.37,50.8 R6.1
DTR
  Top 0.254: R3.1 12.31,21.73 13.08,20.95 Q2.2 13.84,20.83 14.48,20.83 14.99,20.32 14.99,17.27 15.02,17.23 15.02,15.26 16.91,13.38 17.15,13.14 U2.15
ESP-RXD  (via drill 0.35)
  Top 0.254: R38.2 30.46,37.06 v30.05,36.66 | v29.92,21.25 29.26,20.58 26.92,20.58 25.91,19.57 25.91,9.23 25.52,8.84 U7.37
  Bottom 0.254: v30.05,36.66 29.97,36.57 29.97,21.29 v29.92,21.25
ESP-TXD  (via drill 0.35)
  Top 0.254: R25.2 | R25.2 28.7,37.08 v29.12,36.66 | v29.04,21.25 v29.03,21.25 27,21.25 25.5,19.74 25.5,10.5 25.11,10.11 U7.36
  Bottom 0.254: v29.12,36.66 29.21,36.57 29.21,21.42 v29.04,21.25
GND  (via drill 0.35, 0.51 pad 1.02)
  Top 0.254: GND.TP
  Top 0.305: U2.8 12.38,11.84 v12.38,11.87 | U2.20 v19.56,16.39 v19.56,16.38 | USB1.5 4.41,4.42 v4.38,4.45 | U1.2 v67.82,27.94
  Top 0.406: U1.7 U1.2 | U8.4 53.5,20.55 v53.47,20.57
  Top 0.508: ANT1.3 2.09,38.86 0.91,38.86 0.76,38.72 0.76,32.01 0.76,32 v0.76,31.24 | ANT1.2 2.41,44.96 0.76,44.96 0.76,46.2 0.76,47.22 v0.76,48.01 | U7.38 22.67,7.57 v22.67,7.56 | U7.1 38.28,7.56 v36.7,7.56 | U7.15 v36.77,25.46 | C17.1 v42.42,6.03 | C7.1 v40.39,6.03 | C3.1 48.7,7.62 v44.96,7.62 | C4.1 62.36,7.62 v60.96,7.62 | C2.1 v69.34,34.54 | SD1.G1 56.73,35.81 | 56.73,35.81 v58.17,35.81 | 56.73,35.81 v55.37,35.81 | v55.37,50.67 55.31,50.64 SD1.G4 57.91,50.64 v57.91,50.67 | SD1.6 57.91,40.44 v57.91,40.45 | C22.1 C13.1 v43.18,38.86 | C6.1 v42.55,44.9 | v34.67,51.94 U3.1 v34.67,54.23 | C1.1 v36.2,44.9 | C28.1 C27.1 v3.94,13.59 | v6.29,17.72 6.29,17.7 U6.GND 3.49,17.7 v3.49,17.72 | v66.23,52.83 SD1.G3 64.52,51.54 v64.52,51.56 | v64.52,35.81 66.23,35.81 SD1.G2 v66.23,34.54 | USB1.P2 3.17,4.51 v3.17,5.02 | USB1.P1 2.29,6.92 v2.29,7.37 | C21.2 v9.14,21.84 | C20.1 v9.4,26.42 | C18.1 v9.31,4.57 C19.1 | U7.P$1 29.46,15.25 v29.46,14.73 | C24.1 6.04,12.07 R7.1 3.06,12.07 v3.05,12.06 | Q1.2 v43.88,13.91 | R24.1 v44.32,12.19 | C26.1 v62.99,9.91 | R21.1 65.09,9.97 v65.02,9.91 | C23.1 v61.98,25.15 | C25.1 v54.1,30.48 | v15.24,76.96 15.24,72.45 BAT1.- v15.11,67.82 | R20.1 v50.29,20.32 | R11.1 61.53,23.27 v61.55,23.28
  Top 0.61: GND.TP v37.59,38.69 | GND.TP v38.94,37.33 | GND.TP v37.59,35.98 | GND.TP v36.23,37.33
  other vias: 39.12,49.53 39.12,48.26 37.85,48.26 37.85,49.53 36.58,49.53 36.58,48.26 36.58,52.07 37.85,52.07 39.12,52.07 39.12,53.34 37.85,53.34 36.58,53.34 29.97,17.78 28.96,17.78 27.94,17.78 26.92,17.78 32,17.78 30.99,17.78 31.5,16.76 30.48,16.76 29.46,16.76 28.45,16.76 27.43,16.76 26.92,15.75 27.94,15.75 28.96,15.75 29.97,15.75 30.99,15.75 32,15.75 31.5,14.73 30.48,14.73 28.45,14.73 27.43,14.73 26.92,13.72 27.94,13.72 28.96,13.72 29.97,13.72 30.99,13.72 32,13.72 31.5,12.7 30.48,12.7 29.46,12.7 28.45,12.7 27.43,12.7 2.48,2.1 2.98,2.1 2.98,9.33 2.41,9.33 8.64,40.89 12.7,55.37 12.7,42.42 7.87,46.23 7.87,51.05 7.87,52.58 7.87,54.1 7.37,40.89 10.16,40.89 11.43,40.89 12.7,40.89 7.87,44.45 7.87,49.53 9.14,55.37 10.92,55.37 12.7,45.47 12.7,43.94 7.87,48.01 14.22,56.01 16,56.01 13.97,52.58 15.24,52.58 12.7,46.99 12.7,48.51 12.7,50.04 12.7,51.56 2.29,48.01 3.56,48.01 5.08,48.01 6.6,48.01 7.37,39.37 7.37,37.85 7.37,36.32 7.37,34.8 7.37,33.27 7.37,32 2.03,31.24 3.3,31.24 4.83,31.24 6.35,31.24 17.53,56.01 19.05,56.01 20.83,56.01 22.35,56.01 23.88,56.01 24.83,55.24 25.65,54.23 25.65,52.7 25.65,51.18 25.65,49.66 25.65,48.32 23.81,49.66 23.81,48.32 23.81,47.05 25.65,47.05 67.06,30.61 68.58,30.61 68.58,29.84 67.06,29.84 2.22,4.06 3.17,6.48
  pour Top (isolate 0.305): 0,30.48 16.51,30.48 16.51,56.52 0,56.52
  pour Bottom: 0,0 71.12,0 71.12,79.38 0,79.38
  pour Top: 16.51,56.52 28.19,56.52 28.19,30.48 16.51,30.48
GPIO0  (via drill 0.35)
  Top 0.254: Q2.3 11.43,20.32 11.43,24.38 11.94,24.89 19.05,24.89 19.86,24.08 U7.25
  Top 0.305: U7.25 21.49,23.88 22.1,23.88 22.86,23.11 v35.81,23.11 | v49.28,35.56 49.28,36.07 49.77,36.57 R12.1
  Bottom 0.305: v35.81,23.11 36.83,23.11 v49.28,35.56
MICS_PREHEAT_NOX  (via drill 0.35)
  Top 0.305: Q1.1 42.81,15.68 v42.08,16.42 | v39.62,16.42 38.32,16.42 U7.8
  Bottom 0.305: v42.08,16.42 v39.62,16.42
MICS_PWR  (via drill 0.35)
  Top 0.305: Q5.1 44.01,19.62 v42.08,17.69 | v39.79,17.69 38.32,17.69 U7.9
  Bottom 0.305: v42.08,17.69 v39.79,17.69
N$1
  Top 0.254: R16.1 9.2,57.54 3.05,51.39 2.+
N$2
  Top 0.305: R21.2 65.09,13.14 64.01,14.22 62.23,14.22 61.47,14.99 56.13,14.99 55.12,16 U9.C
N$3
  Top 0.305: C5.2 C11.2 C9.1
N$4
  Top 0.305: C9.2 C10.2 ANT1.1
N$5
  Top 0.305: U4.3 14.04,53.68 L1.2 L2.P$1
N$6  (via drill 0.35)
  Top 0.305: U9.A v57.66,15.75 | v48.26,15.75 49.51,15.75
  Top 0.406: 49.51,15.75 R23.2
  Bottom 0.305: v57.66,15.75 v48.26,15.75
N$7
  Top 0.254: 1.+ 4.78,54.4 5.9,55.51 R14.1
N$8
  Top 0.305: L2.P$2 C5.1
N$9
  Top 0.305: U4.5 16.07,54.17 16.51,54.61 22.43,54.61 R6.2
N$10
  Top 0.305: U4.4 15.04,53.66 C15.2 C12.2 21.4,53.66 R5.2
N$11
  Top 0.254: R18.2 17.53,49.28 19.2,47.6 U5.16
N$12
  Top 0.254: Q3.1 16.13,23.62 R3.2
N$13  (via drill 0.35)
  Top 0.254: Q2.1 13.72,18.29 v14.22,17.78 | v17.27,17.53 17.98,18.23 R1.2
  Bottom 0.254: v14.22,17.78 14.48,17.53 v17.27,17.53
N$14
  Top 0.254: R19.2 17.02,47.5 18.1,46.42 U5.17
N$16  (via drill 3.07)
  other vias: 63.5,16.89
N$19  (via drill 3.07)
  other vias: 14.61,3.81
N$20  (via drill 3.07)
  other vias: 67.31,75.56
N$21  (via drill 3.07)
  other vias: 3.81,69.22
N$22
  Top 0.254: 3.+ 7.26,53.83 7.26,54.36 10.31,57.4 R2.1
N$23
  Top 0.305: 47.14,14.77 R24.2 | 47.18,14.73 48.01,14.73 48.67,14.07 R23.1
  Top 0.406: 47.14,14.77 Q1.3 47.18,14.73
N$24
  Top 0.305: Q5.3 50.1,18.73 51.31,17.53 51.31,12.95 52.07,12.19 54.77,12.19 U9.F U9.G U9.H 59.27,12.54 59.84,13.1 U9.J 61.21,13.72 62.23,12.7 C26.2
N$25
  Top 0.508: R7.2 4.44,10.67 4.-
N$26  (via drill 0.35)
  Top 0.305: U2.7 10.83,12.51 10.8,12.48 v9.62,12.48 | USB1.2 4.81,6.37 4.42,6.76 4.42,8.54 4.98,9.1 5.97,9.1 v6.01,9.14
  Bottom 0.305: v6.01,9.14 6.87,9.14 9.62,11.9 v9.62,12.48
N$27  (via drill 0.35)
  Top 0.305: v8.89,13.14 10.34,13.14 U2.6 | USB1.3 4.7,5.71 3.96,6.45 3.96,8.73 5.01,9.78 v6.52,9.78
  Bottom 0.305: v8.89,13.14 8.89,12.06 v6.52,9.78
N$28
  Top 0.254: U2.9 9.92,11.19 9.14,10.41 9.14,7.62 8.3,6.77 | 8.3,6.77 | 8.3,6.77 8.23,6.71 C18.2 7.71,6.1 7.28,5.67 Y1.2
N$29
  Top 0.254: U2.10 10.03,10.54 9.65,10.16 9.65,7.62 10.41,6.86 10.41,6.12 | 10.41,6.12 C19.2 | Y1.1 11.6,5.59 11.07,6.12 10.41,6.12
N$30
  Top 0.254: U2.3 13.87,15.09 16.56,12.39 R34.2
N$33
  Top 0.254: U7.35 20.53,11.38 20.07,10.92 20.07,7.37 19.3,6.6 R33.2
N$36  (via drill 0.35)
  Top 0.254: U6.TXD 6.13,21.45 v6.18,21.5 | R37.2 v14.39,27.01
  Bottom 0.254: v6.18,21.5 6.18,25.21 8.05,27.08 14.32,27.08 v14.39,27.01
N$37
  Top 0.254: R13.1 56.7,4.63 RELOAD.3
N$38
  Top 0.254: RESET.3 44.07,4.45 45.21,3.3 53.09,3.3 53.59,3.81 R4.1
PM_RESET  (via drill 0.35)
  Top 0.254: U6.RESET v6.79,22.7 | v20.15,20.32 20.19,20.27 U7.28
  Bottom 0.254: v6.79,22.7 17.76,22.7 v20.15,20.32
PM_SET  (via drill 0.35)
  Top 0.254: U6.SET 6.08,18.95 v6.09,18.96 | v20.15,18.96 U7.29
  Bottom 0.254: v6.09,18.96 v20.15,18.96
RELOAD  (via drill 0.35)
  Top 0.254: C4.2 64.64,7.75 65.15,7.24 RELOAD.2 | v40.96,11.37 38.3,11.37 U7.4
  Bottom 0.254: RELOAD.2 63.25,3.81 57.66,3.81 54.36,7.11 47.75,7.11 43.5,11.37 v40.96,11.37
RESET  (via drill 0.35)
  Top 0.254: v30.73,10.1 38.27,10.1 U7.3 38.3,10.1 v41.72,10.1 | C3.2 50.93,7.75 51.44,7.24 RESET.2 | 18.29,22.77 19.64,22.77 v19.73,22.77 | 18.29,22.77 | Q3.3 18.29,22.77
  Bottom 0.254: v30.73,10.1 25.46,10.1 21.59,13.97 21.59,21.08 19.89,22.77 v19.73,22.77 | RESET.2 48.39,5.71 44.01,10.1 v41.72,10.1
RF_IN
  Top 0.305: U4.6 15.8,54.67 16.26,55.12 23.62,55.12 24.7,54.04 U5.11
RTS
  Top 0.254: U2.16 17.07,13.79 15.43,15.43 15.43,18.17 R1.1 16.56,20.26 16.17,20.66 Q3.2
RXD0
  Top 0.254: U7.34 20.27,12.65 19.56,11.94 19.56,8.89 19.05,8.38 R34.1
SCL
  Top 0.305: U7.12 40.59,21.54 46.48,27.43 54.86,27.43 57.66,30.23 60.2,30.23 60.72,30.74 R22.1 66.79,31.69 U1.6
SD_CLK_IO14  (via drill 0.35)
  Top 0.305: U7.13 39.32,22.81 39.88,23.37 v39.88,28.19 | v48.07,41.53 R15.1 51.68,41.54 52.32,40.89 54.1,40.89 54.75,41.54 SD1.5
  Bottom 0.305: v39.88,28.19 47.5,35.81 47.5,40.89 48.07,41.47 v48.07,41.53
SD_CMD_IO15  (via drill 0.35)
  Top 0.305: U7.23 25.32,26.34 25.65,26.67 33.19,26.67 34.29,27.77 v34.29,28.19 | v51.82,43.75 R17.1 56.11,43.76 SD1.3
  Bottom 0.305: v34.29,28.19 38.61,28.19 46.74,36.07 46.74,41.97 48.51,43.75 v51.82,43.75
SD_CS_IO13  (via drill 0.35)
  Top 0.305: U7.16 34.21,26.59 v36.07,28.96 | v48.07,44.83 R8.1 SD1.2
  Bottom 0.305: v36.07,28.96 38.61,28.96 45.97,36.32 45.97,42.74 v48.07,44.83
SD_D0_IO2  (via drill 0.35)
  Top 0.305: U7.24 24.05,26.34 25.15,27.43 v32.77,27.43 | SD1.7 56.1,39.37 R9.1 52.59,39.38 51.19,37.98 R12.2 48.97,37.98 v48.96,37.97
  Bottom 0.305: v32.77,27.43 40.13,27.43 48.26,35.56 48.26,37.27 v48.96,37.97
SD_D1_IO4  (via drill 0.35)
  Top 0.305: U7.26 21.49,22.61 22.1,22.61 22.61,22.1 v36.32,22.1 | v54.61,37.34 54.61,37.85 55,38.24 SD1.8
  Bottom 0.305: v36.32,22.1 36.83,22.1 50.29,35.56 53.85,35.56 54.61,36.32 v54.61,37.34
SD_D2_IO12  (via drill 0.35)
  Top 0.305: U7.14 38.28,28.38 v38.29,29.65 | v54.1,45.91 54.13,45.94 SD1.1
  Bottom 0.305: v38.29,29.65 45.21,36.58 45.21,43.56 47.56,45.91 v54.1,45.91
SDA
  Top 0.305: U7.11 40.59,20.27 46.99,26.67 59.69,26.67 60.65,27.63 R10.1 66.79,28.77 U1.1
STAT_LED1  (via drill 0.35)
  Top 0.254: v23.88,59.94 R14.2 | U7.33 22.3,13.92 25.06,16.68 25.06,20.23 v26.16,21.33
  Bottom 0.254: v23.88,59.94 28.45,55.37 28.45,23.62 v26.16,21.33
STAT_LED2  (via drill 0.35)
  Top 0.254: v23.88,58.67 R16.2 | U7.31 22.73,16.46 24.55,18.29 24.55,20.74 v25.14,21.33
  Bottom 0.254: v23.88,58.67 27.69,54.86 27.69,23.88 v25.14,21.33
STAT_LED3  (via drill 0.35)
  Top 0.254: v24.13,57.4 R2.2 | U7.30 23.07,17.73 24.04,18.71 v24.04,21.33
  Bottom 0.254: v24.13,57.4 26.92,54.61 26.92,24.21 v24.04,21.33
TXD0
  Top 0.254: U2.4 13.5,14.44 15.24,12.7 15.24,7.11 15.75,6.6 R33.1
U1RXD  (via drill 0.35)
  Top 0.152: 19.2,39.26 v19.22,39.28 | 28.67,39.28 R25.1
  Top 0.254: U5.3 19.2,39.26 | v25.57,39.28 28.67,39.28
  Bottom 0.254: v19.22,39.28 v25.57,39.28
U1TXD  (via drill 0.35)
  Top 0.152: 18.11,40.54 v18.12,40.55
  Top 0.254: U5.2 18.11,35.54 18.11,40.54 | R38.1 29.25,40.55 v25.57,40.55
  Bottom 0.254: v18.12,40.55 v25.57,40.55
U2RXD  (via drill 0.35)
  Top 0.254: U7.27 v22.69,21.47 | v22.69,27.01 R37.1
  Bottom 0.254: v22.69,21.47 v22.69,27.01
V_BCKP
  Top 0.406: U5.6 22.52,35.81 | 21.84,72.24 BAT1.+2
  Top 0.508: 22.52,35.81 22.52,40.98 23.11,41.57 32.17,41.57 32.17,61.91 21.84,72.24
  Bottom 0.508: BAT1.+1 BAT1.+2
VBUS
  Top 0.305: USB1.1 7.18,7.01 7.79,7.62 L3.1
VCC_RF
  Top 0.305: U5.14 R5.1
VOX_RAWA
  Top 0.305: U9.B 56.39,20.57 55.77,21.2 U8.3 53.74,21.2 53.73,21.21 53.72,21.21 53.2,21.73 R20.2
VOX_RAWB
  Top 0.305: U8.2 U8.1 53.2,22.5 52.83,22.86 48.26,22.86 45.97,20.57 43.69,20.57 41.4,18.28 41.4,16.25 39.07,13.92 U7.6
VRED_RAWA  (via drill 0.35)
  Top 0.305: U9.D 52.94,17.89 v53.59,18.54 | 59.23,19.35 U8.5 61.51,20.55 R11.2
  Top 0.406: v59.18,19.3 59.23,19.35
  Bottom 0.305: v53.59,18.54 54.36,19.3 v59.18,19.3
VRED_RAWB
  Top 0.305: U8.7 U8.6 58.05,21.2 55.88,23.37 48.01,23.37 45.72,21.08 43.18,21.08 40.72,18.62 40.72,16.51 39.39,15.18 38.3,15.18
  Top 0.406: 38.3,15.18 U7.7

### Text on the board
tPlace: Laboratory for Nano-Integrated Systems | Pierre-Emmanuel Gaillardon / Tom Becnel / Trenton Taylor | Support from: | AirU v2.1 / 11/12/18

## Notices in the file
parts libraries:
microbuilder: This work is placed in the public domain, and may be freely used for commercial and non-commercial work with the following conditions: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
